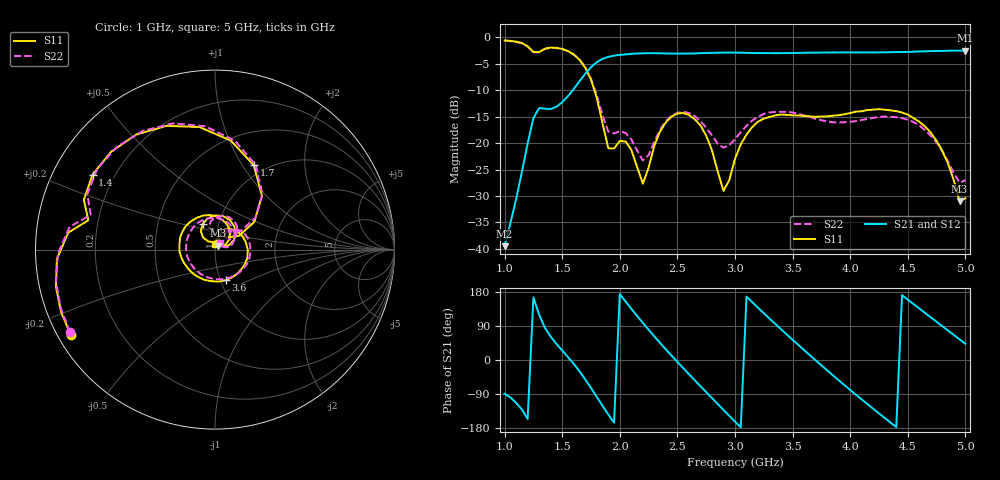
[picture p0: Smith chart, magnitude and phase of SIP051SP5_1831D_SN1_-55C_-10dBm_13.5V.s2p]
# GHz  S  dB  R  50
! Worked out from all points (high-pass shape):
!   81 points, 1 GHz to 5 GHz, reference 50 ohm
!   highest |S21| = -2.50 dB at 5 GHz (marker M1); lowest = -39.5 dB at 1 GHz (marker M2)
!   |S21| within 3 dB of the highest: 1.759 GHz to end of sweep
!   lowest |S11| = -31.0 dB at 4.95 GHz (marker M3), VSWR 1.06, Z = 51.8 + j2.24 ohm
!   |S11| at or under -10 dB: 1.779 GHz to end of sweep
!   |S22| runs from -27.5 to -0.6 dB; largest |S21 - S12| = 0.0019
!   S11 on the Smith chart (normalised r, x): 1 GHz: 0.04, -0.27; 1.4 GHz: 0.12, +0.28; 1.7 GHz: 0.88, +1.13; 2.4 GHz: 0.84, +0.24; 3.6 GHz: 1.06, -0.37; 5 GHz: 1.00, +0.06
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1  -0.59 -149.3  -39.47 -89.2  -39.11 -87.7  -0.63 -150.2
1.25  -2.77 167.2  -15.27 165.1  -15.25 165.2  -2.81 164.7
1.4  -1.94 148.5  -13.56 61.6  -13.55 61.6  -1.99 145.5
1.55  -2.61 111.5  -11.12 7.8  -11.12 7.7  -2.60 108.4
1.7  -5.73 65.3  -6.89 -51.1  -6.88 -51.1  -5.66 64.0
1.85  -16.23 29.9  -4.07 -120.9  -4.08 -121.0  -14.76 36.0
2  -19.59 78.2  -3.33 174.1  -3.33 174.2  -17.77 66.2
2.2  -27.66 94.7  -3.02 97.9  -3.02 98.0  -23.27 76.7
2.35  -17.77 127.7  -3.02 44.9  -3.01 44.9  -17.42 104.6
2.4  -16.06 115.9  -3.05 27.9  -3.04 28.0  -15.80 97.4
2.55  -14.31 77.0  -3.08 -21.2  -3.08 -21.3  -14.08 66.8
2.75  -18.59 27.0  -2.97 -84.8  -2.96 -84.8  -17.10 33.9
2.9  -29.03 40.9  -2.89 -131.8  -2.89 -131.8  -20.86 43.2
3  -22.97 83.8  -2.90 -162.6  -2.89 -162.5  -19.25 56.5
3.3  -15.05 13.5  -2.98 109.2  -3.00 109.2  -14.20 16.9
3.6  -14.86 -70.9  -2.92 26.1  -2.94 26.1  -14.75 -49.6
3.7  -15.03 -97.2  -2.90 -0.8  -2.90 -0.8  -15.39 -76.7
4.05  -14.04 -177.1  -2.85 -91.6  -2.84 -91.7  -15.85 177.9
4.35  -13.80 119.5  -2.82 -165.1  -2.82 -165.1  -15.00 97.8
4.7  -18.03 48.4  -2.61 112.4  -2.61 112.5  -18.59 25.4
4.95  -30.98 49.8  -2.52 54.3  -2.52 54.3  -27.52 31.4
5  -30.39 88.1  -2.50 42.8  -2.51 42.7  -27.00 50.9
